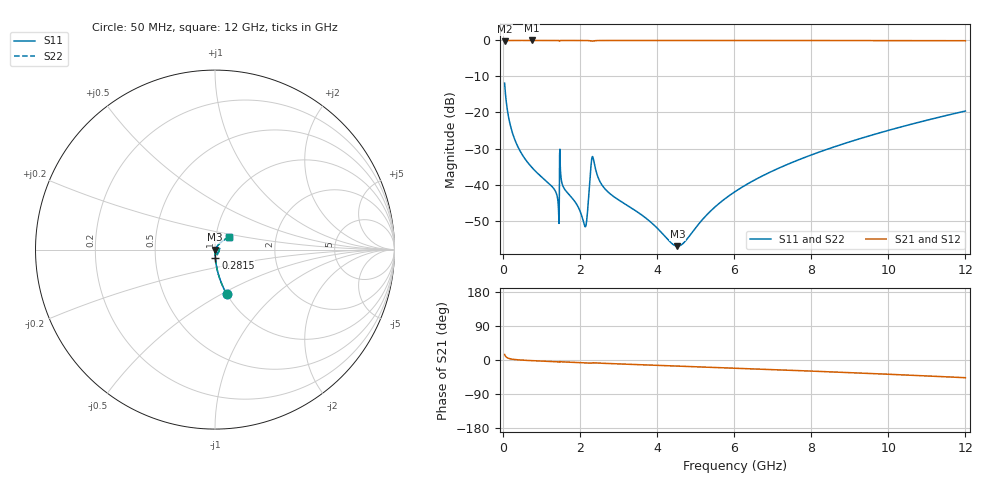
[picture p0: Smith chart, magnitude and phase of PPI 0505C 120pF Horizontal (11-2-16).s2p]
# MHz S MA R 50
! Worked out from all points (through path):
!   1601 points, 50 MHz to 12 GHz, reference 50 ohm
!   highest |S21| = -0.01 dB at 752.1 MHz (marker M1); lowest = -0.3 dB at 50 MHz (marker M2)
!   group delay of S21, straight-line fit = 11 ps
!   lowest |S11| = -57.1 dB at 4.531 GHz (marker M3), VSWR 1.00, Z = 50.1 - j0.0446 ohm
!   |S11| at or under -10 dB: start of sweep to end of sweep
!   |S22| runs from -57.1 to -11.8 dB; largest |S21 - S12| = 0
!   S11 on the Smith chart (normalised r, x): 50 MHz: 1.00, -0.53; 281.5 MHz: 1.00, -0.09; 12 GHz: 1.16, +0.16
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50  0.2557 -75.3  0.9665 14.6  0.9665 14.6  0.2557 -75.3
162.0312  0.08131 -85.7  0.9963 4.1  0.9963 4.1  0.08131 -85.7
281.5312  0.04688 -87.8  0.9985 1.7  0.9985 1.7  0.04688 -87.8
475.7188  0.02771 -89.0  0.9991 -0.1  0.9991 -0.1  0.02771 -89.0
752.0625  0.01741 -89.6  0.9992 -1.7  0.9992 -1.7  0.01741 -89.6
1297.281  0.009164 -88.9  0.999 -4.1  0.999 -4.1  0.009164 -88.9
1409.312  0.007018 -86.4  0.9989 -4.6  0.9989 -4.6  0.007018 -86.4
1536.281  0.01052 -89.7  0.9989 -4.9  0.9989 -4.9  0.01052 -89.7
1596.031  0.008805 -89.4  0.999 -5.2  0.999 -5.2  0.008805 -89.4
2044.156  0.003764 -74.0  0.9984 -7.0  0.9984 -7.0  0.003764 -74.0
2118.844  0.002723 -49.5  0.9978 -7.4  0.9978 -7.4  0.002723 -49.5
2163.656  0.002781 -14.8  0.9971 -7.6  0.9971 -7.6  0.002781 -14.8
2290.625  0.01828 2.8  0.9819 -8.3  0.9819 -8.3  0.01828 2.8
2350.375  0.02292 -52.1  0.9834 -7.4  0.9834 -7.4  0.02292 -52.1
2507.219  0.01143 -85.1  0.9972 -8.2  0.9972 -8.2  0.01143 -85.1
2686.469  0.008331 -88.3  0.9982 -9.0  0.9982 -9.0  0.008331 -88.3
4038.312  0.002392 -70.4  0.9984 -14.1  0.9984 -14.1  0.002392 -70.4
4531.25  0.001397 -18.6  0.9983 -16.0  0.9983 -16.0  0.001397 -18.6
6025  0.00797 56.7  0.998 -21.6  0.998 -21.6  0.00797 56.7
8019.156  0.02594 56.3  0.9972 -29.3  0.9972 -29.3  0.02594 56.3
10013.31  0.05668 49.9  0.9953 -37.7  0.9953 -37.7  0.05668 49.9
12000  0.1049 41.6  0.9907 -46.8  0.9907 -46.8  0.1049 41.6
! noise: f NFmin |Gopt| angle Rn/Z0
50  0.0003444  0.8482  0.3836  0.0004827
1372  0.003583  0.6441  4.914  0.001903
2701  0.006525  0.6217  9.618  0.003199
4031  0.007567  0.5403  14.25  0.002878
5360  0.009365  0.5172  18.78  0.003307
6682  0.01118  0.5046  23.18  0.003768
8012  0.01305  0.4988  27.45  0.004268
9341  0.01501  0.4986  31.57  0.004825
1.067e+04  0.0171  0.503  35.53  0.00546
1.2e+04  0.01937  0.5116  39.32  0.006203
